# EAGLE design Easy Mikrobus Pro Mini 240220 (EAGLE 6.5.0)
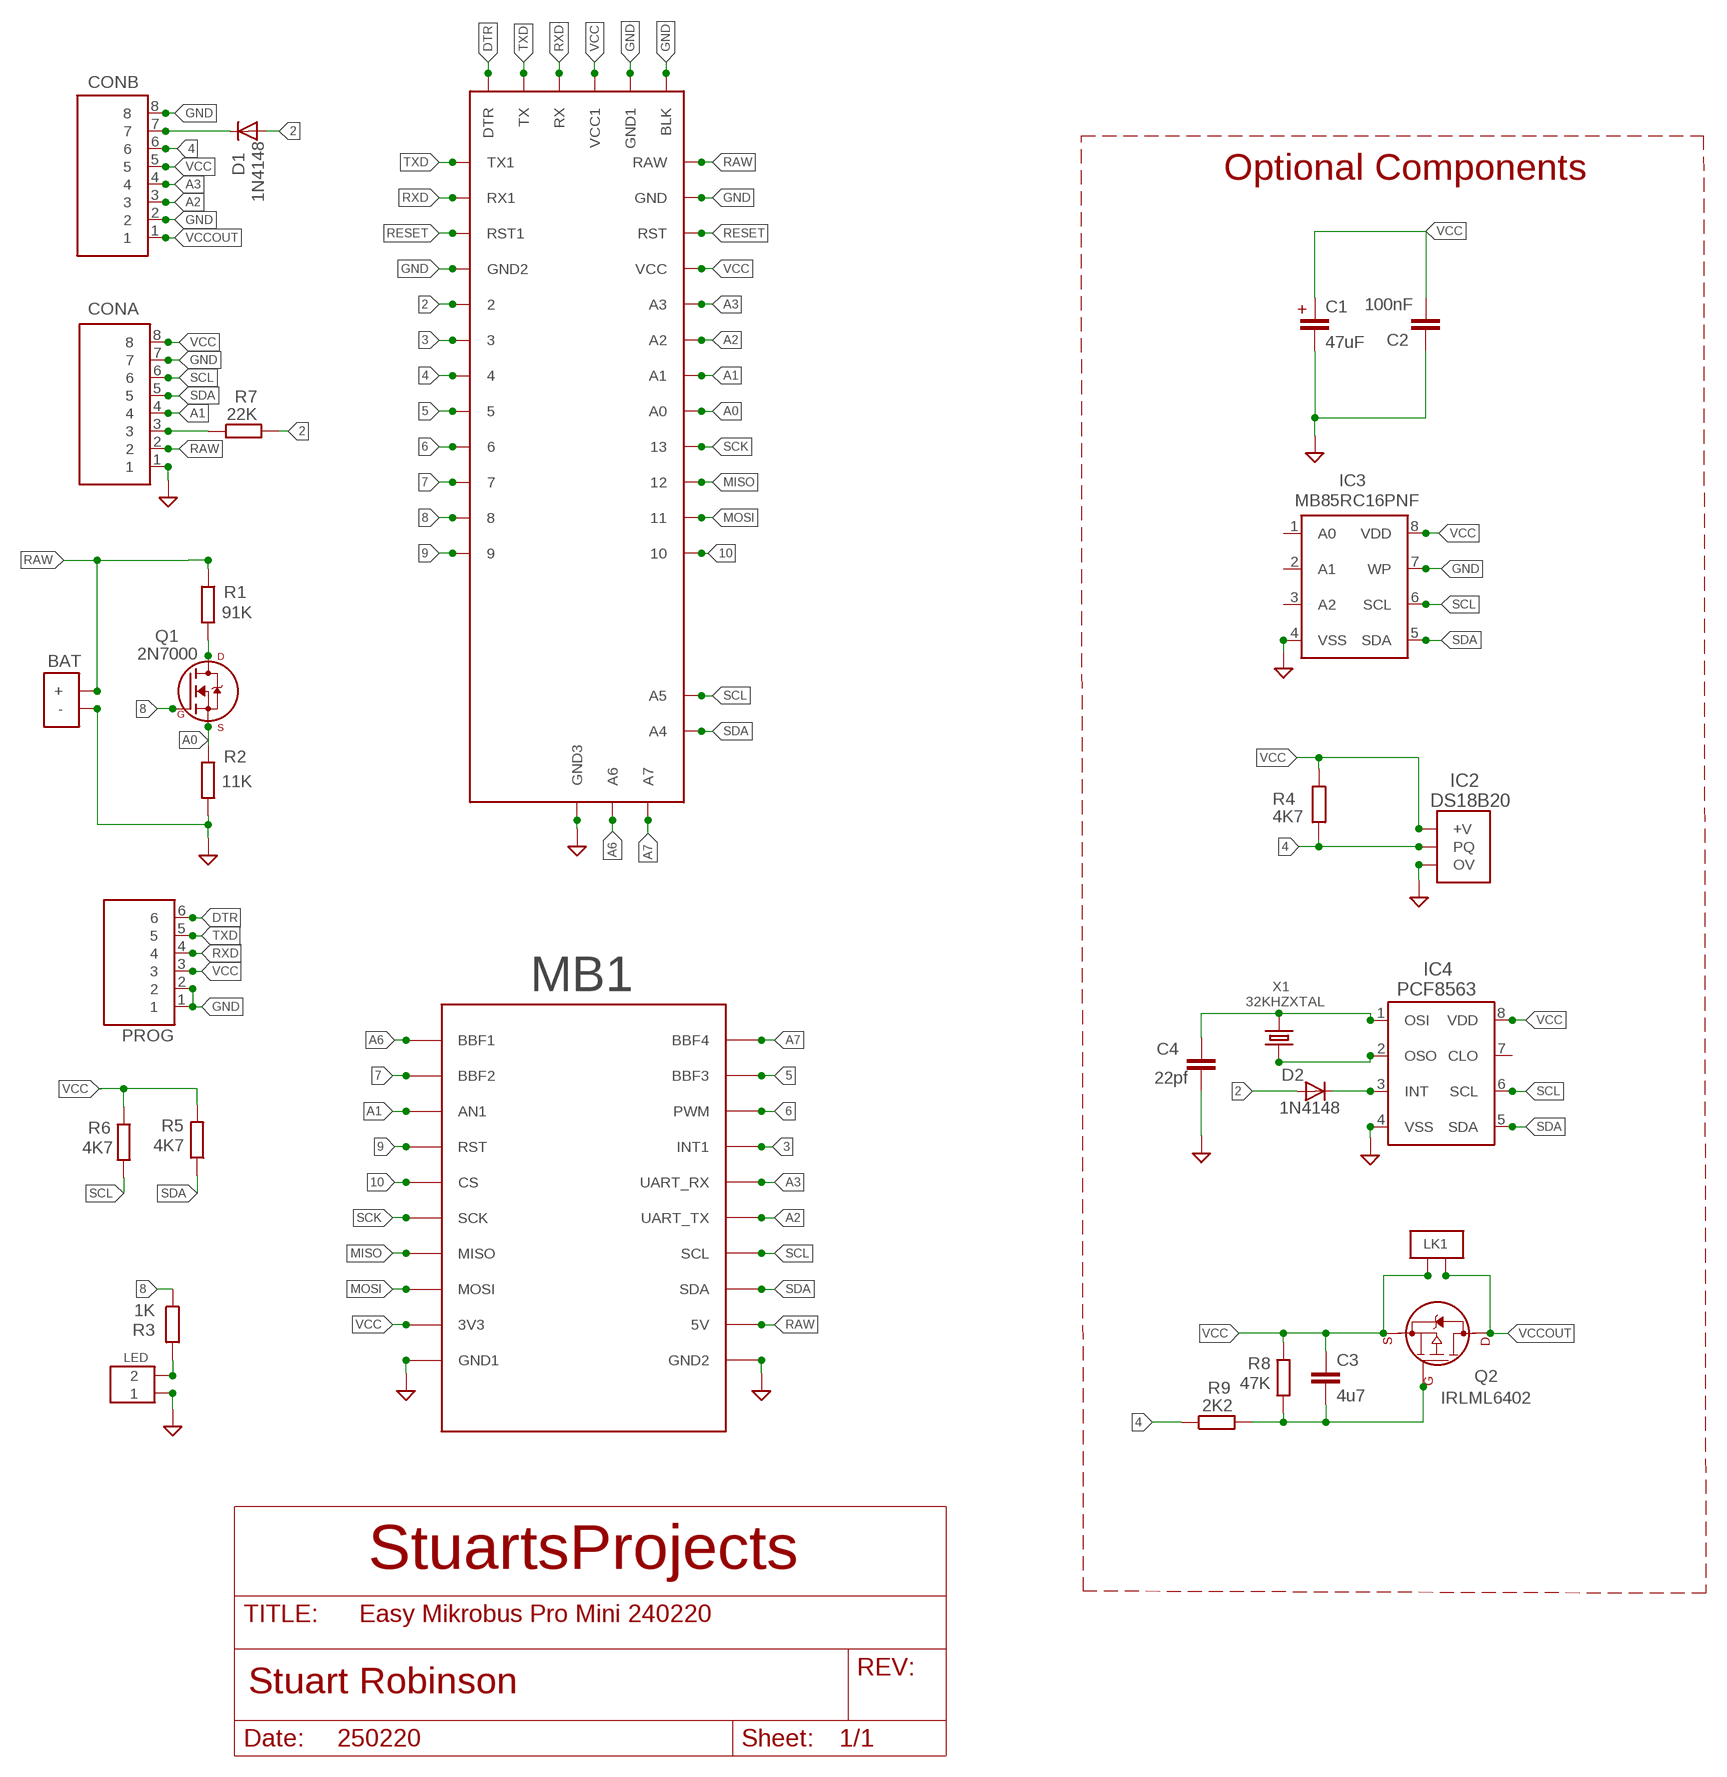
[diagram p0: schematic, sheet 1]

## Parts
BAT  BATPADS2  [BATPADS]
C1  47uF  2.5MM_SPACEING_CAPACITOR  [2.5MM_SPACING_CAPACITOR]
C2  100nF  AXIAL_CERAMICDEFAULT  [AXIAL_CERAMIC]
C3  4u7  C-EUC1206  [C1206]
C4  22pf  C2,5-3  [C2.5-3]
CONA  8X1  [8X1]
CONB  8X1  [8X1]
D1  1N4148  SIGNAL_DIODE  [SIGNAL_DIODE]
D2  1N4148  SIGNAL_DIODE  [SIGNAL_DIODE]
IC1  PROMINIV2  [PROMINI_HEADER2]
IC2  DS18B20  [TO92]
IC3  MB85RC16PNF  24L256SOIC2  [SOIC_2]
IC4  PCF8563  [SOIC08@1]
LED  2PIN  [2PIN]
LK1  BYPASS_LINKMEDIUM2  [BYPASS_LINK_MEDIUM1]
MB1  BBFRIENDY2  [PCB_SOCKET_BBFRIENDLY2]
PROG  6X1  [6X1]
Q1  2N7000  [T092_MIN]
Q2  IRLML6402  IRLFL6402  [SOT23@1]
R1  91K  125MWRESISTOR  [125MWRESISTOR]
R2  11K  125MWRESISTOR  [125MWRESISTOR]
R3  1K  125MWRESISTOR  [125MWRESISTOR]
R4  4K7  125MWRESISTOR  [125MWRESISTOR]
R5  4K7  125MWRESISTOR  [125MWRESISTOR]
R6  4K7  125MWRESISTOR  [125MWRESISTOR]
R7  22K  125MWRESISTOR  [125MWRESISTOR]
R8  47K  R-EU_M1206  [M1206]
R9  2K2  R-EU_M1206  [M1206]
X1  32KHZXTAL  [32KHZXTAL]

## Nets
2: D1.A D2.A IC1.2 R7.P$2
3: IC1.3 MB1.INT(INT1)
4: CONB.6 IC1.4 IC2.2(PQ) R4.P$2 R9.1
5: IC1.5 MB1.BBF3
6: IC1.6 MB1.PWM
7: IC1.7 MB1.BBF2
8: IC1.8 Q1.2(G) R3.P$1
9: IC1.9 MB1.RST
10: IC1.10 MB1.CS
A0: IC1.A0 Q1.1(S) R2.P$1
A1: CONA.4 IC1.A1 MB1.AN1
A2: CONB.3 IC1.A2 MB1.TX(UART_TX)
A3: CONB.4 IC1.A3 MB1.RX(UART_RX)
A6: IC1.A6 MB1.BBF1
A7: IC1.A7 MB1.BBF4
DTR: IC1.DTR PROG.6
GND [POWER]: BAT.BAT-V(-) C1.- C2.P$2 C4.1 CONA.1 CONA.7 CONB.2 CONB.8 IC1.BLK IC1.GND IC1.GND1 IC1.GND2 IC1.GND_3(GND3) IC2.1(OV) IC3.4(VSS) IC3.7(WP) IC4.4(VSS) LED.P$1 MB1.GND1(GND2) MB1.GND2(GND1) PROG.1 PROG.2 R2.P$2
MISO: IC1.12 MB1.MISO
MOSI: IC1.11 MB1.MOSI
N$1: Q1.3(D) R1.P$2
N$2: LED.P$2 R3.P$2
N$3: CONB.7 D1.C
N$4: CONA.3 R7.P$1
N$5: D2.C IC4.3(INT)
N$8: C3.2 Q2.1(G1) R8.1 R9.2
N$11: C4.2 IC4.1(OSI) X1.P$2
N$12: IC4.2(OSO) X1.P$3
RAW [POWER]: BAT.BAT+(+) CONA.2 IC1.RAW MB1.5V R1.P$1
RESET: IC1.RST IC1.RST1
RXD: IC1.RX IC1.RX1 PROG.4
SCK: IC1.13 MB1.SCK
SCL: CONA.6 IC1.A5 IC3.6(SCL) IC4.6(SCL) MB1.SCL R6.P$1
SDA: CONA.5 IC1.A4 IC3.5(SDA) IC4.5(SDA) MB1.SDA R5.P$1
TXD: IC1.TX IC1.TX1 PROG.5
VCC [VDD]: C1.+ C2.P$1 C3.1 CONA.8 CONB.5 IC1.VCC IC1.VCC1 IC2.3(+V) IC3.8(VDD) IC4.8(VDD) LK1.P$2 MB1.3V3 PROG.3 Q2.2(S1) R4.P$1 R5.P$2 R6.P$2 R8.2
VCCOUT [VDD]: CONB.1 LK1.P$1 Q2.3(D1)
Unconnected: IC3.1(A0) IC3.2(A1) IC3.3(A2) IC4.7(CLO)

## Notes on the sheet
- Optional Components
- StuartsProjects
- 250220

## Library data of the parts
BAT = LMA2:BATPADS2
C1 = LMA2:2.5MM_SPACEING_CAPACITOR
C2 = LMA2:AXIAL_CERAMIC
C3 = resistor:C-EU: CAPACITOR, European symbol
C4 = capacitor-wima:C: CAPACITOR
CONA CONB = My_Pin_Headers:8X1
D1 D2 = LMA2:SIGNAL_DIODE
IC1 = LMA2:PROMINIV2
IC2 = LMA2:DS18B20
IC3 = LMA2:24L256
IC4 = LMA2:PCF8563
LED = LMA2:2PIN
LK1 = LMA2:BYPASS_LINK
MB1 = My_Mikrobus:BBFRIENDY2
PROG = My_Pin_Headers:6X1
Q1 = LMA:2N7000
Q2 = LMA2:IRLFL6402
R1-R7 = LMA2:125MWRESISTOR
R8 R9 = resistor:R-EU_: RESISTOR, European symbol
X1 = LMA2:32KHZXTAL

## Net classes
0 default: width 0.152 mm
1 POWER: width 0.559 mm
2 VDD: width 0.559 mm
3 gpspower: width 0.559 mm

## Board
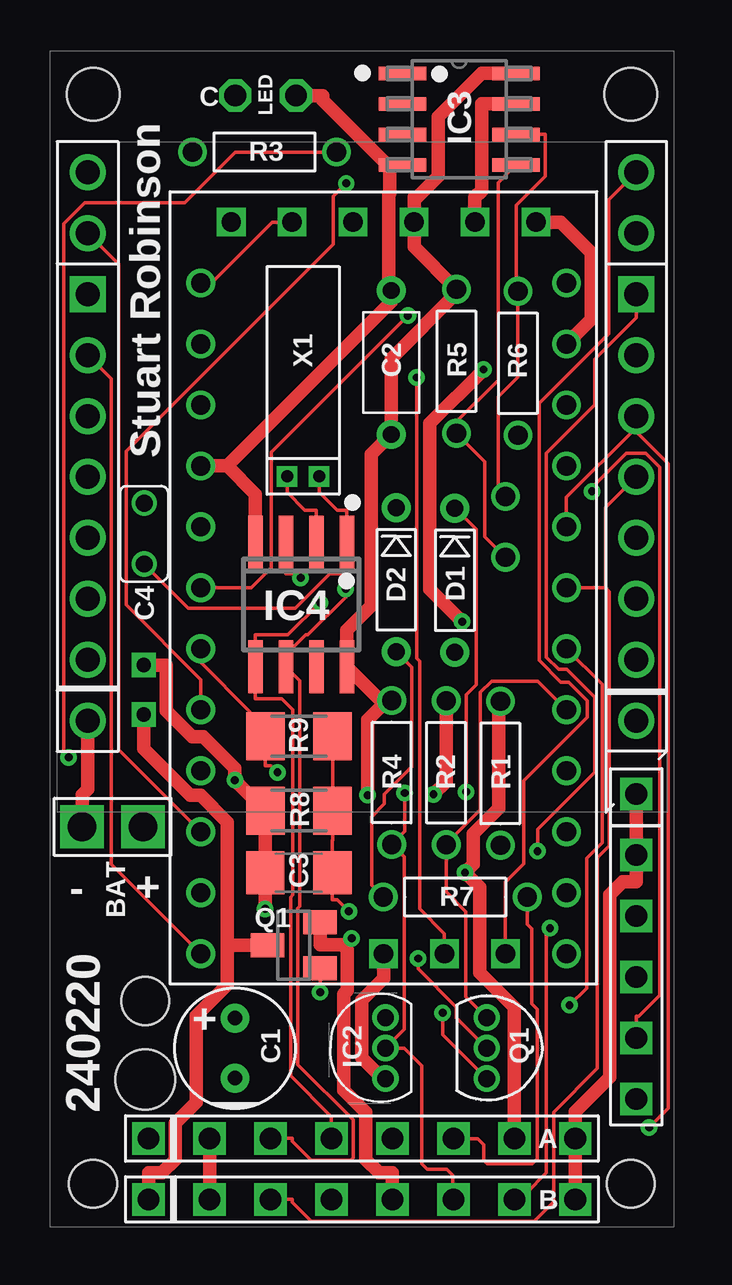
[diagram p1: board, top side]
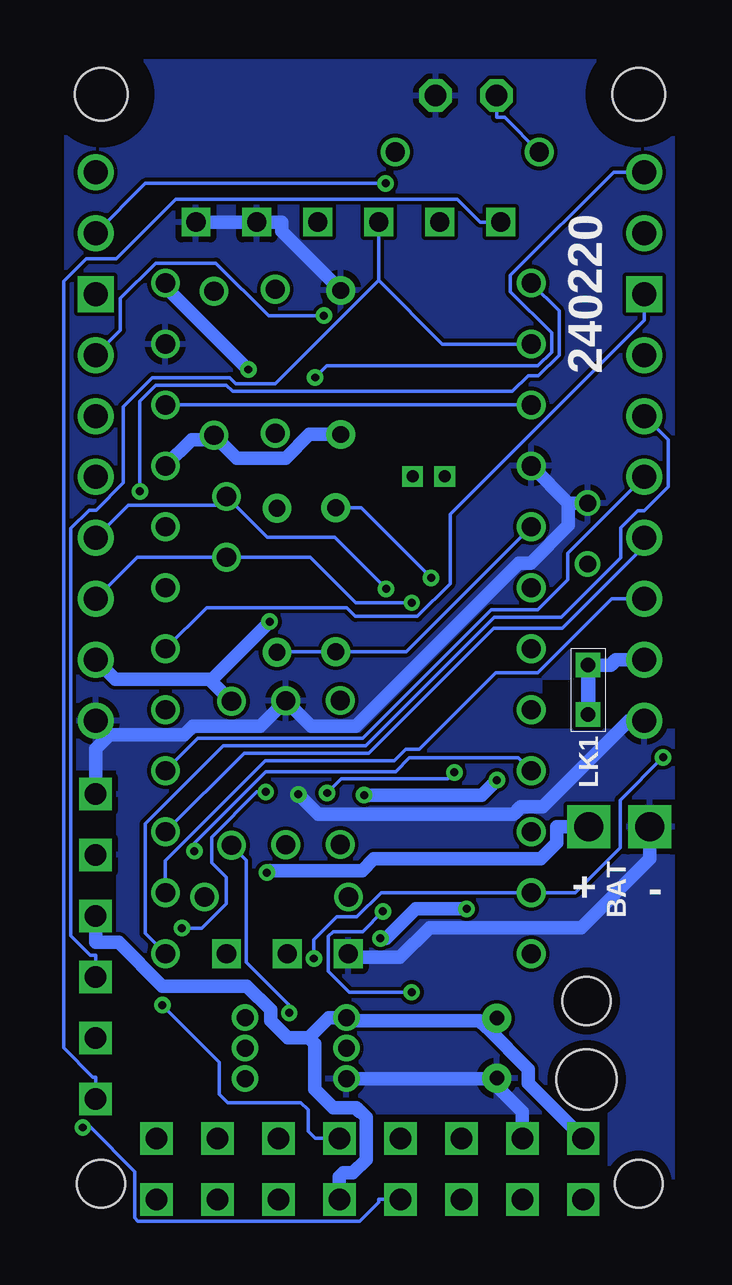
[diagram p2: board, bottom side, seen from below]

No outline drawn. Coordinates in mm, seen from the top.
Copper layers (1*16): Top 0.0356mm / dielectric 1.5011mm / Bottom 0.0356mm
Design rules "LaenPCBOrder *": minimum track width 6mil, minimum drill 13mil, track to track 6mil, track to pad 6mil, pad to pad 6mil, via to via 6mil, smd to smd 6mil, copper to edge 15mil, drill to drill 6mil, minimum pad ring 7mil, minimum via ring 7mil, stop-mask expansion 4mil, vias tented up to drill 1000mil, thermal gap 10mil
Holes 2.2 mm at 1.8,47.2 24.2,47.2
Holes 2 mm at 1.8,1.8 24.2,1.8 3.97,9.41
Holes 2.5 mm at 3.97,6.15
tRestrict: area 22.2,45.2 to 26.2,49.2; area -0.2,45.2 to 3.8,49.2
bRestrict: area -0.2,45.2 to 3.8,49.2; area 22.2,45.2 to 26.2,49.2; area 25.8,0 to 26,49; area 0,0 to 0.3,49; area 0,0 to 26,0.2; area 3.1,0.2 to 22.9,4.7; area 0,48.7 to 26,49; area 0.3,21.9 to 5.8,22.8; area 0.3,20.8 to 6.2,21.9; area 23.6,4.2 to 25.2,19

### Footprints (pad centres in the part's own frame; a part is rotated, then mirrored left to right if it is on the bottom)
BATPADS = drill 1.2 pad 1.778 square: BAT+ 0,-1.27; BAT-V 0,1.27
2.5MM_SPACING_CAPACITOR = drill 0.6 pad 1.2: + 0,1.25; - 0,-1.25
AXIAL_CERAMIC = drill 0.7 pad 1.2: P$1 -3,0; P$2 3,0
C1206 = smd 1.6 x 1.8: 1 -1.4,0; 2 1.4,0
C2.5-3 = drill 0.7: 1 -1.27,0; 2 1.27,0
8X1 = drill 0.9 square: 1 -8.89,0; 2 -6.35,0; 3 -3.81,0; 4 -1.27,0; 5 1.27,0; 6 3.81,0; 7 6.35,0; 8 8.89,0
SIGNAL_DIODE = drill 0.7 pad 1.2: A -3,0; C 3,0
PROMINI_HEADER2 = drill 0.8: 2 -7.62,19.05; 3 -7.62,16.51; 4 -7.62,13.97; 5 -7.62,11.43; 6 -7.62,8.89; 7 -7.62,6.35; 8 -7.62,3.81; 9 -7.62,1.27; 10 7.62,1.27; 11 7.62,3.81; 12 7.62,6.35; 13 7.62,8.89; A0 7.62,11.43; A1 7.62,13.97; A2 7.62,16.51; A3 7.62,19.05; A4 5.08,17.78; A5 5.08,20.32; GND 7.62,26.67; GND2 -7.62,21.59; RAW 7.62,29.21; RST 7.62,24.13; RST1 -7.62,24.13; RX1 -7.62,26.67; TX1 -7.62,29.21; VCC 7.62,21.59 | drill 0.8 square: A6 2.54,1.27; A7 5.08,1.27; BLK 6.35,31.75; DTR -6.35,31.75; GND1 3.81,31.75; GND_3 0,1.27; RX -1.27,31.75; TX -3.81,31.75; VCC1 1.27,31.75
TO92 = drill 0.7 pad 1.1: 1 -1.27,0.07; 2 0,0.07; 3 1.27,0.07
SOIC_2 = smd 1.981 x 0.559: 1 -2.362,1.905; 2 -2.362,0.635; 3 -2.362,-0.635; 4 -2.362,-1.905; 5 2.362,-1.905; 6 2.362,-0.635; 7 2.362,0.635; 8 2.362,1.905
SOIC08@1 = smd 0.6 x 2.2: 1 -1.905,-2.6; 2 -0.635,-2.6; 3 0.635,-2.6; 4 1.905,-2.6; 5 1.905,2.6; 6 0.635,2.6; 7 -0.635,2.6; 8 -1.905,2.6
2PIN = drill 0.9 octagon: P$1 0,1.27; P$2 0,-1.27
BYPASS_LINK_MEDIUM1 = drill 0.6 pad 1.016 square: P$1 -1.03,0; P$2 1.03,0
PCB_SOCKET_BBFRIENDLY2 = drill 1: 3V3 -11.43,5.08; 5V 11.43,5.08; BBF1 -11.43,25.4; BBF2 -11.43,22.86; BBF3 11.43,22.86; BBF4 11.43,25.4; CS -11.43,15.24; GND1 -11.43,2.54; GND2 11.43,2.54; INT 11.43,17.78; MISO -11.43,10.16; MOSI -11.43,7.62; RST -11.43,17.78; RX 11.43,15.24; SCK -11.43,12.7; SCL 11.43,10.16; SDA 11.43,7.62; TX 11.43,12.7 | drill 1 square: AN1 -11.43,20.32; PWM 11.43,20.32
6X1 = drill 0.9 square: 1 -6.35,0; 2 -3.81,0; 3 -1.27,0; 4 1.27,0; 5 3.81,0; 6 6.35,0
T092_MIN = drill 0.7 pad 1.1: 1 -1.27,0; 2 0,0; 3 1.27,0
SOT23@1 = smd 1 x 1.4: 1 -0.95,-1.1; 2 0.95,-1.1; 3 0,1.1
125MWRESISTOR = drill 0.8: P$1 -3,0 | drill 0.8 pad 1.2: P$2 3,0
M1206 = smd 1.6 x 2: 1 -1.4,0; 2 1.4,0
32KHZXTAL = drill 0.5 pad 0.711 square: P$2 -6.75,-0.667; P$3 -6.75,0.667

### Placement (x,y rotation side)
BAT  2.61,16.67 90 top
C1  7.71,7.45 0 top
C2  14.22,36.02 90 top
C3  10.37,14.76 0 top
C4  3.93,28.89 270 top
CONA  13,3.69 180 top
CONB  13,1.15 0 top
D1  16.87,26.95 90 top
D2  14.43,26.97 90 top
IC1  13.9,10.12 0 top
IC2  14.05,7.45 90 top
IC3  17.05,46.16 0 top
IC4  10.47,25.94 180 top
LED  8.99,47.14 270 top
LK1  3.91,22.38 90 bottom
MB1  13,18.55 0 top
PROG  24.43,11.69 270 top
Q1  18.2,7.45 270 top
Q2  10.16,11.74 90 top
R1  18.77,18.9 270 top
R2  16.51,18.93 90 top
R3  8.94,44.79 180 top
R4  14.24,18.94 270 top
R5  16.94,36.07 90 top
R6  19.5,35.99 270 top
R7  16.89,13.75 180 top
R8  10.38,17.35 180 top
R9  10.38,20.45 0 top
X1  10.55,38.02 90 top

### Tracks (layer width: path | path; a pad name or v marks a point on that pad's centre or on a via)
2
  Top 0.152: D2.A 15.07,23.33 15.07,19.18 13.93,18.04 13.93,17.62 13.4,17.1 13.4,14.24 R7.P$2
  Bottom 0.152: IC1.2 11.48,23.97 D2.A 16.84,23.97 D1.A
3  (via drill 0.33 pad 0.69)
  Top 0.152: v14.92,37.97 9.23,32.28 9.23,27.47 8.39,26.63 IC1.3
  Bottom 0.152: MB1.INT 23.4,37.36 23.4,38.69 21.93,40.16 19.41,40.16 17.22,37.97 v14.92,37.97
4  (via drill 0.33 pad 0.69)
  Top 0.152: v9.48,18.94 9.2,19.22 8.98,19.22 8.98,19.84 R9.1 8.33,21.1 8.33,21.47 6.28,23.52 6.28,23.81 IC1.4 | v14.78,18.08 14.78,16.48 R4.P$2 14.76,15.42 14.76,8.23 IC2.2 14.76,7.45 15.5,6.71 15.5,2.64 15.73,2.41 16.54,2.41 16.79,2.16 16.79,1.17 CONB.6
  Bottom 0.152: v14.78,18.08 14.19,18.67 9.75,18.67 v9.48,18.94
5  (via drill 0.33 pad 0.69)
  Top 0.152: IC1.5 6.28,22.81 3.17,25.92 3.17,32.32 11.8,40.95 11.8,42.94 v12.35,43.49
  Bottom 0.152: v12.35,43.49 22.35,43.49 MB1.BBF3
6  (via drill 0.33 pad 0.69)
  Top 0.152: MB1.PWM 24.43,37.89 22.7,36.16 22.7,34.26 20.69,32.24 20.69,23.75 21.19,23.24 21.53,23.24 22.7,22.07 22.7,18.95 20.32,16.57 v20.32,15.66
  Bottom 0.152: v20.32,15.66 20.32,15.99 17.33,18.98 11.93,18.98 11.36,19.55 6.82,19.55 IC1.6
7
  Top 0.152: MB1.BBF2 2.87,40.11 2.87,19.88 IC1.7
8  (via drill 0.33 pad 0.69)
  Top 0.152: Q1.2 16.93,8.72 16.93,9.16 15.34,10.76 v15.34,11.19 | R3.P$1 7.73,44.79 5.62,42.68 1.46,42.68 0.58,41.81 0.58,19.76 v0.78,19.56
  Bottom 0.152: v15.34,11.19 15.34,11.98 14.39,12.92 13.55,12.92 12.54,13.93 IC1.8 4.45,13.93 2.57,15.81 2.57,17.79 0.8,19.56 v0.78,19.56
9
  Top 0.152: MB1.RST 2.56,35.34 2.56,15.11 IC1.9
10
  Bottom 0.152: IC1.10 22.37,12.24 22.37,16.8 19.11,20.05 13.17,20.05 7.81,25.41 5.03,25.41 2.55,27.89 2.55,29.14 1.85,29.84 1.57,29.84 0.57,30.84 0.57,32.79 MB1.CS
A0
  Top 0.152: Q1.1 17.33,9.59 17.33,13.14 16.51,13.96 R2.P$1 16.51,15.97 17.93,17.39 17.93,22.27 18.4,22.75 20.32,22.75 IC1.A0
A1  (via drill 0.33 pad 0.69)
  Top 0.152: v21.65,9.24 22.36,9.96 22.36,15.36 23.01,16.01 23.01,22.6 IC1.A1
  Bottom 0.152: MB1.AN1 1.57,37.79 9.66,29.69 9.66,26.8 11.02,25.44 13.61,25.44 13.97,25.8 19.81,25.8 IC1.A1 | v21.65,9.24 19.27,6.87 19.27,6.12 19.27,5.53 18.92,5.18 15.88,5.18 15.58,4.88 15.58,3.99 15.28,3.69 CONA.4
A2
  Top 0.152: 23.16,26.63 23.31,26.48 23.31,15.88 22.82,15.39 22.82,6.61 20.99,4.78 20.99,1.06 20.18,0.25 10.88,0.25 10.09,1.04 10.09,1.15 CONB.3 | 23.16,26.63 IC1.A2 | MB1.TX 23.16,29.98 23.16,26.63
A3  (via drill 0.33 pad 0.69)
  Top 0.152: 24.34,33.21 25.76,31.79 25.76,4.94 v24.96,4.15 | MB1.RX 24.43,33.3 24.34,33.21 | 24.34,33.21 21.52,30.39 IC1.A3
  Bottom 0.152: CONB.4 12.63,1.15 12.63,1.04 13.43,0.25 22.66,0.25 22.79,0.38 22.79,2.31 24.63,4.15 v24.96,4.15
A6  (via drill 0.33 pad 0.69)
  Top 0.152: v15.28,35.4 15.28,23.69 15.41,23.57 15.41,13.25 16.44,12.22 IC1.A6
  Bottom 0.152: MB1.BBF1 2.84,43.95 7.14,39.65 7.14,38.97 5.42,37.25 5.42,36.46 6,35.88 14.79,35.88 v15.28,35.4
A7
  Top 0.152: MB1.BBF4 23.29,42.81 23.29,37.23 20.38,34.32 20.38,23.61 21.29,22.7 21.62,22.7 22.39,21.92 22.39,21.25 19.74,18.6 19.74,15.14 18.98,14.37 IC1.A7
DTR
  Bottom 0.152: IC1.DTR 8.38,41.87 8.41,41.87 9.36,42.82 21.09,42.82 23.57,40.34 24.82,40.34 25.76,39.4 25.76,7.46 24.54,6.24 24.43,6.24 PROG.6
GND  (via drill 0.33 pad 0.69)
  Top 0.559: R2.P$2 16.51,18.56 v15.98,18.03 | LED.P$1 11.37,47.14 11.37,46.95 14.06,44.26 | 14.06,44.26 14.16,44.15 14.16,43.08 14.11,43.02 14.11,39.13 C2.P$2 14.22,38.54 7.39,31.71 | BAT.BAT-V 1.34,18 1.57,18.23 MB1.GND1 | IC2.1 13.86,6.18 13,7.04 13,9.46 13.9,10.36 IC1.GND_3 | IC3.4 14.06,44.26 | 7.39,31.71 8.56,30.53 8.56,30.07 IC4.4 | IC1.GND2 7.39,31.71 | CONB.8 CONA.1 21.89,4.24 21.89,4.8 23.32,6.23 23.32,13.84 23.88,14.39 24.43,14.39 PROG.2 PROG.1 | IC1.GND1 17.71,42.9 17.99,43.18 17.99,46.8 IC3.7 | IC1.BLK 21.28,41.87 22.56,40.59 22.56,37.83 IC1.GND | CONB.2 CONA.7
  Bottom 0.559: v15.98,18.03 15.16,17.21 7,17.21 6.71,17.5 5.81,17.5 2.22,21.09 MB1.GND1 | 4.73,30.16 4.73,29.23 6.3,27.66 6.8,27.66 13.59,20.87 15.45,20.87 R2.P$2 17.57,20.87 20.38,20.87 20.74,20.51 23.85,20.51 | BAT.BAT-V 1.34,15.34 4.2,12.48 10.51,12.48 11.76,11.23 13.74,11.23 IC1.GND_3 | 23.85,20.51 MB1.GND2 | PROG.1 24.43,19.93 23.85,20.51 | IC1.BLK IC1.GND1 16.68,41.87 16.68,41.48 C2.P$2 | CONA.7 6.65,4.8 7.73,5.88 7.73,6.18 | IC2.1 7.73,6.18 | 7.73,6.18 C1.- | C4.1 4.73,30.16 | 4.73,30.16 IC1.GND2
  pour Bottom: 0,49 26,49 26,0 0,0
MISO
  Bottom 0.152: IC1.12 18.24,19.75 13.04,19.75 7.84,24.95 4.98,24.95 1.57,28.37 MB1.MISO
MOSI
  Bottom 0.152: IC1.11 21.52,15.27 17.37,19.42 11.98,19.42 11.5,19.9 10.95,19.9 7.75,23.1 6,23.1 2.93,26.17 2.83,26.17 MB1.MOSI
N$1  (via drill 0.33 pad 0.69)
  Top 0.152: v16.36,8.92 16.36,8.02 Q1.3
  Bottom 0.152: R1.P$2 18.15,15.28 18.15,11.03 16.36,9.24 v16.36,8.92
N$2
  Bottom 0.152: LED.P$2 7.72,46.24 7.39,46.24 R3.P$2
N$3  (via drill 0.33 pad 0.69)
  Top 0.152: D1.C 17.76,29.06 17.76,22.59 17.34,22.17 v17.34,18.13 | v20.84,12.45 20.68,12.3 20.68,2.82 20.68,2.4 20.68,2.25 19.86,1.43 19.63,1.43 CONB.7
  Bottom 0.152: v20.84,12.45 20.01,12.45 18.99,13.47 18.99,14.58 19.6,15.19 19.6,16.25 17.72,18.13 v17.34,18.13
N$4
  Top 0.152: 20.3,2.86 20.3,2.84 20.1,2.64 | 20.1,2.64 18.22,2.64 18.08,2.78 18.08,3.43 17.83,3.68 CONA.3 | 20.1,2.64 20.31,2.85 20.31,9.07 20.07,9.31 20.07,12.43 19.89,12.61 19.89,13.73 19.9,13.8 R7.P$1
N$5  (via drill 0.33 pad 0.69)
  Top 0.152: IC4.3 9.84,27.21 10.28,27.21 v10.45,27.05
  Bottom 0.152: D2.C 13.37,29.97 v10.45,27.05
N$8  (via drill 0.33 pad 0.69)
  Top 0.152: R9.2 R8.1 11.78,16.12 11.77,16.11 C3.2 11.77,13.63 11.98,13.63 v12.46,13.15 | Q2.1 v11.26,9.78
  Bottom 0.152: v12.46,13.15 13.3,12.31 14.52,12.31 14.73,12.11 14.73,10.65 13.85,9.78 v11.26,9.78
N$11
  Top 0.152: X1.P$2 11.22,30.61 11.96,29.87 12.38,29.87 IC4.1 12.38,27.21 11.65,27.21 10.22,25.78 5.77,25.78 C4.2
N$12
  Top 0.152: IC4.2 11.11,29.87 10.63,29.87 9.88,30.61 X1.P$3
RAW  (via drill 0.33 pad 0.69)
  Top 0.559: v17.18,25.22 15.82,26.58 15.82,33.48 v18.07,35.73 | CONA.2 19.35,9.15 17.9,10.6 17.9,14.16 v17.3,14.76 17.64,15.11 17.64,16.39 18.7,17.45 18.7,21.7 R1.P$1
  Bottom 0.559: 19.58,22.82 v17.18,25.22 | MB1.5V 23.62,22.82 19.58,22.82 | R1.P$1 19.58,22.71 19.58,22.82 | IC1.RAW 21.52,39.18 v18.07,35.73 | BAT.BAT+ 5.21,16.67 5.21,16 5.88,15.34 12.83,15.34 13.33,14.84 17.22,14.84 v17.3,14.76
RESET
  Bottom 0.152: IC1.RST1 IC1.RST
RXD
  Bottom 0.152: 12.63,39.44 IC1.RX | 12.63,39.44 16.94,35.12 18.59,35.12 18.85,35.39 22.06,35.39 23.28,34.17 23.28,31 24.41,29.87 24.7,29.87 25.46,29.12 25.46,12.12 24.66,11.32 24.43,11.32 PROG.4 | IC1.RX1 9.98,36.79 12.63,39.44
SCK
  Bottom 0.152: IC1.13 20.17,20.36 13.3,20.36 7.94,25.72 6,25.72 4.75,26.97 4.75,28.07 MB1.SCK
SCL  (via drill 0.33 pad 0.69)
  Top 0.152: v12.32,26.59 12.32,26.25 10.75,24.68 10.67,24.68 9.84,23.84 IC4.6 10.42,22.76 10.42,13.37 10.33,13.29 10.33,6.77 12.63,4.47 12.63,2.89 12.53,2.79 10.88,2.79 10.09,3.58 10.09,3.69 CONA.6 | IC1.A5 18.67,30.75 18.67,34.59 19.5,35.41 R6.P$1 19.42,39.07 19.42,42.57 20.63,43.78 20.63,45.52 IC3.6
  Bottom 0.152: v12.32,26.59 14.46,28.73 17.27,28.73 IC1.A5 19.34,30.08 23.06,30.08 MB1.SCL
SDA  (via drill 0.33 pad 0.69)
  Top 0.152: v11.26,26.01 9.92,24.67 8.56,24.67 IC4.5 8.56,22.01 9.65,22.01 10.11,21.55 10.11,13.83 10.03,13.75 10.03,6.3 11.73,4.59 CONA.5 | IC3.5 18.67,43.51 18.67,35.29 16.94,33.56 R5.P$1 18.12,31.89 18.12,28.76 IC1.A4
  Bottom 0.152: v11.26,26.01 13.6,26.01 15.49,27.9 IC1.A4 22.7,27.9 MB1.SDA
TXD  (via drill 0.33 pad 0.69)
  Top 0.152: IC1.TX 9.26,41.87 6.72,39.33 IC1.TX1 | PROG.5 24.43,8.78 24.54,8.78 25.42,9.66 25.42,31.65 24.83,32.24 24.02,32.24 22.59,30.81 v22.59,30.65
  Bottom 0.152: IC1.TX1 5.12,38.17 5.12,36.33 5.98,35.47 6.41,35.47 7.06,34.82 18.72,34.82 18.98,35.08 21.91,35.08 22.59,34.41 v22.59,30.65
VCC  (via drill 0.33 pad 0.69)
  Top 0.559: v8.97,13.25 C3.1 8.97,15.91 8.98,15.92 R8.2 v7.71,18.62 7.71,19.11 6.39,20.43 5.93,20.43 4.85,21.52 4.85,23.41 LK1.P$2 | 13.91,21.8 13.24,21.12 v13.24,18 | 12.24,11.71 12.19,11.76 11.26,11.76 Q2.2 | 12.24,11.71 12.39,11.56 12.39,9.86 12.24,9.7 12.24,5.7 13.16,4.77 13.16,2.81 13.72,2.26 14.27,2.26 CONB.5 | 12.24,11.71 v12.57,12.03 | 13.91,21.8 IC4.8 12.38,24.87 13.39,25.89 13.39,32.19 C2.P$1 14.22,36.17 16.94,38.9 R5.P$2 15.17,40.84 IC1.VCC1 15.17,42.9 15.3,42.9 16.18,43.78 16.18,46.26 17.99,48.06 IC3.8 | 13.91,21.8 14.05,21.94 R4.P$1
  Bottom 0.559: 15.55,7.89 16.43,7.89 17.14,8.6 17.14,9.04 18.12,10.03 21.65,10.03 23.47,11.85 24.43,11.85 PROG.3 | v7.71,18.62 8.33,18 v13.24,18 | v12.57,12.03 12.31,12.03 11.09,13.25 v8.97,13.25 | 8.12,8.29 8.42,8.6 13.86,8.6 IC2.3 14.15,8.72 14.72,8.72 15.55,7.89 | CONB.5 14.27,2.09 14.11,2.26 13.72,2.26 13.16,2.81 13.16,4.57 13.39,4.8 13.42,4.8 13.58,4.96 14.52,4.96 15.29,5.73 15.29,7.63 15.55,7.89 | LK1.P$2 2.97,23.41 2.75,23.63 MB1.3V3 | IC1.VCC 20.43,32.8 19.7,32.8 R6.P$2 18.55,32.04 16.51,32.04 15.53,33.02 | C2.P$1 15.53,33.02 | 15.53,33.02 | 8.12,8.29 C1.+ | CONA.8 6.4,5.98 6.4,6.57 8.12,8.29
  Bottom 0.61: LK1.P$2 3.91,21.37
VCCOUT
  Top 0.559: CONB.1 4.11,2.26 4.66,2.26 5.22,2.81 5.22,4.32 6.1,5.2 6.1,8.8 7.39,10.09 7.39,11.74 | 7.39,11.74 7.39,16.86 6.28,17.98 5.85,17.98 3.91,19.92 LK1.P$1 | Q2.3 7.39,11.74

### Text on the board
tPlace: LED | C | IC3 | R3 | C2 | R5 | R6 | X1 | Stuart Robinson | D2 | D1 | C4 | IC4 | R9 | R2 | R1 | R4 | R8 | BAT | - | + | C3 | Q1 | R7 | C1 | IC2 | Q1 | 240220 | A | B
bPlace: 240220 | LK1 | BAT | + | -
